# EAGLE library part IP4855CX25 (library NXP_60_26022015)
SD 3.0-compliant memory card integrated voltage level translator with EMI filter and ESD protection The device is an SD 3.0-compliant 6-bit bidirectional dual voltage level translator. It is designed to interface between a memory card operating at 1.8 V or 2.9 V signal levels and a host with a fixed nominal supply voltage of 1.2 V to 3.3 V. The device supports SD 3.0 SDR50, DDR50, SDR25, SDR12 and SD 2.0 High-Speed (50 MHz) and Default-Speed (25 MHz) modes. The device has an integrated switchable voltage regulator to supply the card-side I/Os, built-in EMI filters and robust ESD protections (IEC 61000-4-2, level 4). AAL Eindhoven MK
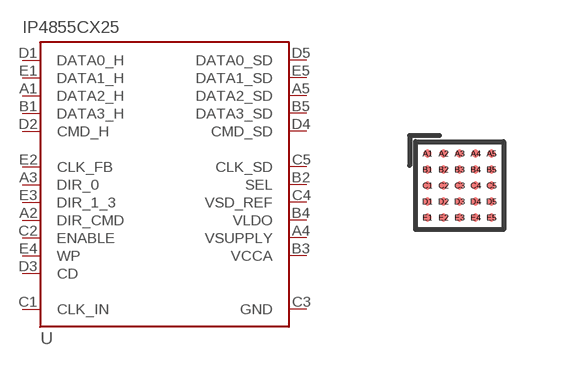
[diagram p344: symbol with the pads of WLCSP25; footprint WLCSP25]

Designator prefix U

## IP4855CX25  [WLCSP25]
A1  DATA2_H
A2  DIR_CMD
A3  DIR_0
A4  VSUPPLY  pwr
A5  DATA2_SD
B1  DATA3_H
B2  SEL
B3  VCCA  pwr
B4  VLDO  pwr
B5  DATA3_SD
C1  CLK_IN
C2  ENABLE
C3  GND  pwr
C4  VSD_REF
C5  CLK_SD  out
D1  DATA0_H
D2  CMD_H
D3  CD
D4  CMD_SD
D5  DATA0_SD
E1  DATA1_H
E2  CLK_FB  out
E3  DIR_1_3
E4  WP
E5  DATA1_SD

## Footprint WLCSP25 (pad centres in mm)
WLCSP25 Wafer level chip-size package; 25 bumps (5 x 5) JEDEC: -- IEC: -- JEITA: --
smd 0.2 x 0.2: A1 -0.8,0.8; A2 -0.4,0.8; A3 0,0.8; A4 0.4,0.8; A5 0.8,0.8; B1 -0.8,0.4; B2 -0.4,0.4; B3 0,0.4; B4 0.4,0.4; B5 0.8,0.4; C1 -0.8,0; C2 -0.4,0; C3 0,0; C4 0.4,0; C5 0.8,0; D1 -0.8,-0.4; D2 -0.4,-0.4; D3 0,-0.4; D4 0.4,-0.4; D5 0.8,-0.4; E1 -0.8,-0.8; E2 -0.4,-0.8; E3 0,-0.8; E4 0.4,-0.8; E5 0.8,-0.8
